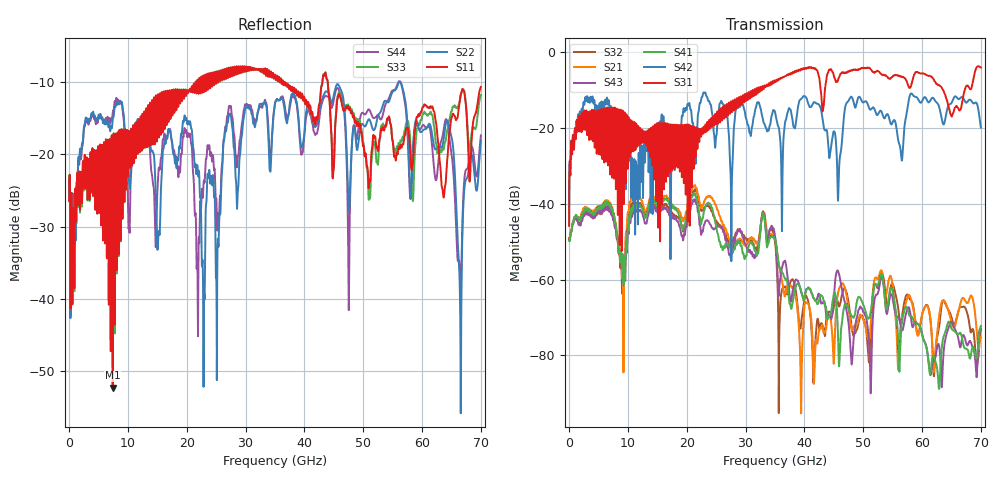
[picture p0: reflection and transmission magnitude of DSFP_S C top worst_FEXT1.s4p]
! AWR Design Environment (8415) Wed Jan 09 11:11:49 2019
! Document = 'DSFP_S'
! nPorts: 4, nXvals: 7001
# HZ S DB R 50
!Freq DBS11 AngS11 DBS12 AngS12 DBS13 AngS13 DBS14 AngS14
!	DBS21 AngS21 DBS22 AngS22 DBS23 AngS23 DBS24 AngS24
!	DBS31 AngS31 DBS32 AngS32 DBS33 AngS33 DBS34 AngS34
!	DBS41 AngS41 DBS42 AngS42 DBS43 AngS43 DBS44 AngS44
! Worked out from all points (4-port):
!   7000 points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, 10 MHz to 70 GHz, reference 50 ohm
!   strongest paths, dB at 10 MHz, 17.51 GHz, 35.01 GHz, 52.51 GHz, 70 GHz:
!     S31: -45.8, -28.1, -7.6, -5.0, -4.0
!     S42: -45.6, -25.7, -15.8, -16.4, -19.9
!     S41: -49.7, -40.3, -49.5, -61.3, -72.3
!     S43: -49.4, -43.0, -48.5, -63.6, -73.2
!     S21: -49.3, -40.1, -49.2, -59.8, -75.2
!     S32: -49.0, -42.3, -50.1, -62.1, -72.9
!   lowest |S11| = -52.2 dB at 7.42 GHz (marker M1), VSWR 1.00, Z = 50 + j0.24 ohm
!   |S11| at or under -10 dB: start of sweep to 21.5 GHz; 36.64 GHz to 43.07 GHz (6.432 GHz wide, 16.1 % of centre); 43.96 GHz to end of sweep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
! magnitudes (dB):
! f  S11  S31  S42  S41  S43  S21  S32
! 10 MHz  -26.4  -45.8  -45.6  -49.7  -49.4  -49.3  -49.0
! 7.42 GHz  -52.2  -15.4  -15.0  -42.3  -43.7  -42.1  -43.6
! 22.82 GHz  -9.1  -20.3  -10.7  -42.8  -46.2  -40.1  -41.6
! 33.11 GHz  -8.5  -9.4  -18.7  -43.1  -42.7  -42.2  -42.6
! 39.42 GHz  -12.2  -4.4  -12.3  -62.8  -63.0  -93.1  -72.0
! 66.46 GHz  -12.3  -15.2  -12.1  -74.0  -77.9  -66.7  -67.3
! 70 GHz  -10.7  -4.0  -19.9  -72.3  -73.2  -75.2  -72.9
